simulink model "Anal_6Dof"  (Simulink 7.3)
settings: Solver=ode45  StartTime=0.0  StopTime=500  RelTol=1e-3
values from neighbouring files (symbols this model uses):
  calfa = cos(alfa0*d2r)    [run.m]
  d2r = pi/180    (= 0.0174532925199)    [run.m]
  klr = [0.82083770557  -0.70145835124   0.75722294555   0.32691190448   0.14993771995;        0.55253708187   0.66141640307  -0.4963339086    0.20601876795  -0.07844376733]    [run.m]
  kls = [0.23009875115  -1.3857134134    0.5565800989    0.03843893525  0.1360972015;        0.22658853965   0.3268097242   -0.0904376422    0.0272194403  -0.00768778705]    [run.m]
  r2d = 180/pi    (= 57.2957795131)    [Pl.m]    (also in run.m)
  salfa = sin(alfa0*d2r)    [run.m]
  Thet0 = 43    [run.m]
  V0 = 18640    [run.m]
undefined symbols (not defined in the file or in its folder): A6d, B6d, C6d, D6d, KJmix, KSmix

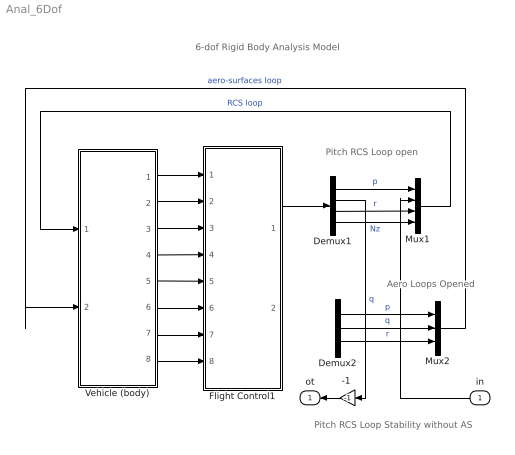
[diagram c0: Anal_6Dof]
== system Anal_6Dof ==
  note: 6-dof Rigid Body Analysis Model
  note: Pitch RCS Loop open
  note: Aero Loops Opened
  note: Pitch RCS Loop Stability without AS
  in : Inport  OutDataType=sfix(16)  OutScaling=2^0
  "-1 " : Gain  Gain=-1  ParameterDataType=sfix(16)  ParameterScaling=2^0  OutDataType=sfix(16)  OutScaling=2^0
  Demux1 : Demux
  Demux2 : Demux  Outputs=3
  Flight Control1 : Subsystem
  Mux1 : Mux
  Mux2 : Mux  Inputs=3
  Vehicle (body) : Subsystem
  ot : Outport  OutDataType=sfix(16)  OutScaling=2^0
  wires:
  Mux2/1 -> Vehicle (body)/2(Aer_pqr)  "aero-surfaces loop"
  Vehicle (body)/2(p) -> Flight Control1/2(pb)
  Vehicle (body)/3(r) -> Flight Control1/3(rb)
  Vehicle (body)/6(q) -> Flight Control1/6(q)
  Vehicle (body)/5(thet) -> Flight Control1/5(thet)
  Vehicle (body)/7(alf) -> Flight Control1/7(alfa)
  Vehicle (body)/4(bet) -> Flight Control1/4(beta)
  Vehicle (body)/1(phi) -> Flight Control1/1(phi)
  Vehicle (body)/8(Nz) -> Flight Control1/8(Nz)
  "-1 "/1 -> ot/1
  Mux1/1 -> Vehicle (body)/1(Jet_pqr)  "RCS loop"
  Demux1/4 -> Mux1/4  "Nz"
  Demux1/3 -> Mux1/3  "r"
  Demux1/1 -> Mux1/1  "p"
  Demux2/1 -> Mux2/1  "p"
  Demux2/3 -> Mux2/3  "r"
  Flight Control1/1(Jet_pqr) -> Demux1/1
  Demux2/2 -> Mux2/2  "q"
  Demux1/2 -> "-1 "/1  "q"
  in/1 -> Mux1/2

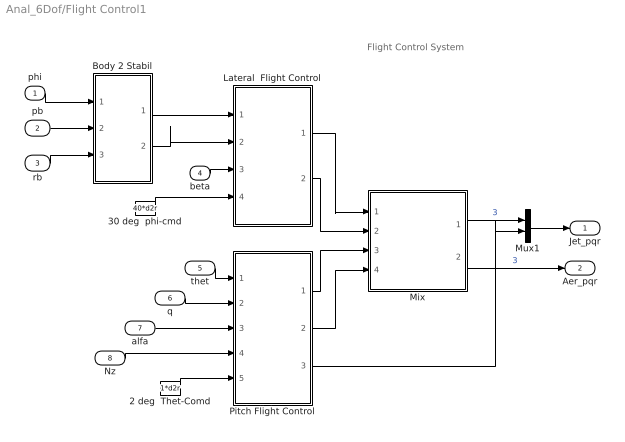
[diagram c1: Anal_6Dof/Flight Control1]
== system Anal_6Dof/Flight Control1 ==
  note: Flight Control System
  phi : Inport  OutDataType=sfix(16)  OutScaling=2^0
  pb : Inport  Port=2  OutDataType=sfix(16)  OutScaling=2^0
  rb : Inport  Port=3  OutDataType=sfix(16)  OutScaling=2^0
  beta : Inport  Port=4  OutDataType=sfix(16)  OutScaling=2^0
  thet : Inport  Port=5  OutDataType=sfix(16)  OutScaling=2^0
  q : Inport  Port=6  OutDataType=sfix(16)  OutScaling=2^0
  alfa : Inport  Port=7  OutDataType=sfix(16)  OutScaling=2^0
  Nz : Inport  Port=8  OutDataType=sfix(16)  OutScaling=2^0
  2 deg  Thet-Comd : Constant  Value=1*d2r  OutDataType=sfix(16)  OutScaling=2^0
  30 deg  phi-cmd : Constant  Value=40*d2r  OutDataType=sfix(16)  OutScaling=2^0
  Body 2 Stabil : Subsystem
  Lateral  Flight Control : Subsystem
  Mix : Subsystem
  Mux1 : Mux  Inputs=[3,1]
  Pitch Flight Control : Subsystem
  Jet_pqr : Outport  OutDataType=sfix(16)  OutScaling=2^0
  Aer_pqr : Outport  Port=2  OutDataType=sfix(16)  OutScaling=2^0
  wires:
  Lateral  Flight Control/1(rcs_PR) -> Mix/1(Rcs_PR)
  Lateral  Flight Control/2(aero_PR) -> Mix/2(Aer_PR)
  Pitch Flight Control/1(rcs_Q) -> Mix/3(Rcs_Q)
  Pitch Flight Control/2(aero_Q) -> Mix/4(Aer_Q)
  beta/1 -> Lateral  Flight Control/3(beta)
  Mix/2(Aer_pqr) -> Aer_pqr/1  "3"
  thet/1 -> Pitch Flight Control/1(thet)
  q/1 -> Pitch Flight Control/2(q)
  alfa/1 -> Pitch Flight Control/3(alf)
  Body 2 Stabil/2(r_s) -> Lateral  Flight Control/2(rs)
  Body 2 Stabil/1(p_s) -> Lateral  Flight Control/1(ps)
  rb/1 -> Body 2 Stabil/3(r_b)
  pb/1 -> Body 2 Stabil/2(p_b)
  phi/1 -> Body 2 Stabil/1(phi)
  Nz/1 -> Pitch Flight Control/4(Nz)
  Mix/1(Jet_pqr) -> Mux1/1  "3"
  2 deg  Thet-Comd/1 -> Pitch Flight Control/5(alf-cmd)
  30 deg  phi-cmd/1 -> Lateral  Flight Control/4(phi-cmd)
  Pitch Flight Control/3(Nzfb) -> Mux1/2
  Mux1/1 -> Jet_pqr/1

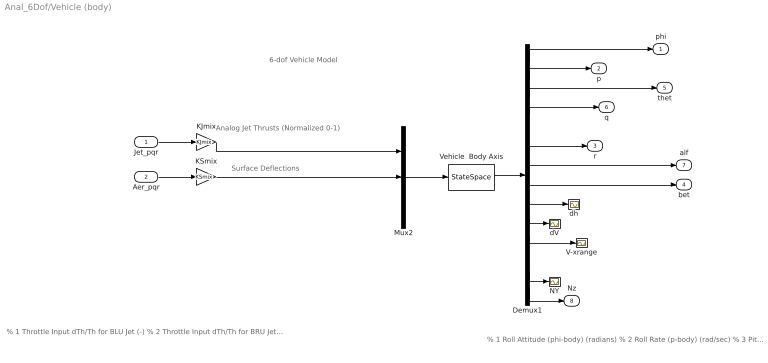
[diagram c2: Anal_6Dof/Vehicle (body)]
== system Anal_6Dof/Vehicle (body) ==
  note: 6-dof Vehicle Model
  note: % 1 Throttle Input dTh/Th for BLU Jet (-) % 2 Throttle Input dTh/Th for BRU Jet (-) % 3 Throttle Input dTh/Th for BLD Jet (-) % 4 Throttle Input dTh/Th for BRD Jet (-) % 5 Throttle Input dTh/Th for BL+Y Jet (-) % 6 Throttle Input dTh/Th for BR-Y Jet (-) % 7 Throttle Input dTh/Th for FU Jet (-) % 8 Throttle Input dTh/Th for FD Jet (-) % 9 Throttle Input dTh/Th for FL Jet (-) % 10 Throttle Input dTh/Th for FR Jet (-) % 11 Left Outbrd Elevon Deflection (radians) % 12 Left Inboard Elevon Deflection (radians) % 13 Right Inbrd Elevon Deflection (radians) % 14 Right Outbrd Elevon Deflection (radians) % 15 Vertical Rudder Deflection (radians) % 16 Gust Veloc, Azim-Elev Angles=(45,90) (deg)
  note: % 1 Roll Attitude (phi-body) (radians) % 2 Roll Rate (p-body) (rad/sec) % 3 Pitch Attitude (thet-bdy) (radians) % 4 Pitch Rate (q-body) (rad/sec) % 5 Yaw Attitude (psi-body) (radians) % 6 Yaw Rate (r-body) (rad/sec) % 7 Angle of attack, alfa, (radians) % 8 Angle of sideslip, beta, (radian) % 9 Change in Altitude, delta-h, (feet) % 10 Forward Acceleration (V-dot) (ft/sec) % 11 Cross Range Velocity (Vcr) (ft/sec) % 12 CG Acceleration along X axis, (ft/sec^2) % 13 CG Acceleration along Y axis, (ft/sec^2) % 14 CG Acceleration along Z axis, (ft/sec^2)
  note: Analog Jet Thrusts (Normalized 0-1)
  note: Surface Deflections
  Jet_pqr : Inport  OutDataType=sfix(16)  OutScaling=2^0
  Aer_pqr : Inport  Port=2  OutDataType=sfix(16)  OutScaling=2^0
  Demux1 : Demux  Outputs=14
  KJmix : Gain  Gain=KJmix  Multiplication=Matrix(K*u)  ParameterDataType=sfix(16)  ParameterScaling=2^0  OutDataType=sfix(16)  OutScaling=2^0
  KSmix : Gain  Gain=KSmix  Multiplication=Matrix(K*u)  ParameterDataType=sfix(16)  ParameterScaling=2^0  OutDataType=sfix(16)  OutScaling=2^0
  Mux2 : Mux  Inputs=[11, 5, 1]
  NY : Scope
  V-xrange : Scope
  Vehicle  Body Axis : StateSpace  A=A6d  B=B6d  C=C6d  D=D6d
  dV : Scope
  dh : Scope
  phi : Outport  OutDataType=sfix(16)  OutScaling=2^0
  p : Outport  Port=2  OutDataType=sfix(16)  OutScaling=2^0
  r : Outport  Port=3  OutDataType=sfix(16)  OutScaling=2^0
  bet : Outport  Port=4  OutDataType=sfix(16)  OutScaling=2^0
  thet : Outport  Port=5  OutDataType=sfix(16)  OutScaling=2^0
  q : Outport  Port=6  OutDataType=sfix(16)  OutScaling=2^0
  alf : Outport  Port=7  OutDataType=sfix(16)  OutScaling=2^0
  Nz : Outport  Port=8  OutDataType=sfix(16)  OutScaling=2^0
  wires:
  Demux1/11 -> V-xrange/1
  Demux1/13 -> NY/1
  Demux1/14 -> Nz/1
  Demux1/10 -> dV/1
  Demux1/9 -> dh/1
  Vehicle  Body Axis/1 -> Demux1/1
  Demux1/1 -> phi/1
  Demux1/3 -> thet/1
  Aer_pqr/1 -> KSmix/1
  Jet_pqr/1 -> KJmix/1
  Demux1/8 -> bet/1
  Demux1/7 -> alf/1
  Demux1/6 -> r/1
  Demux1/4 -> q/1
  Demux1/2 -> p/1
  KJmix/1 -> Mux2/1
  KSmix/1 -> Mux2/2
  Mux2/1 -> Vehicle  Body Axis/1

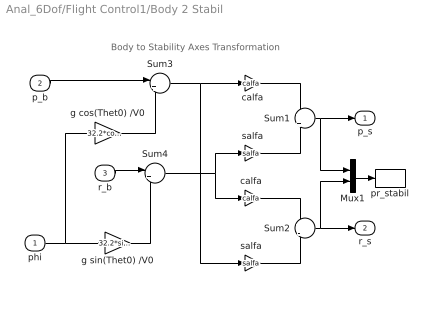
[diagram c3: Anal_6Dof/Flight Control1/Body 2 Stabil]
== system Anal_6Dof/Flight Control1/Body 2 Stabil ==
  note: Body to Stability Axes Transformation
  phi : Inport  OutDataType=sfix(16)  OutScaling=2^0
  p_b : Inport  Port=2  OutDataType=sfix(16)  OutScaling=2^0
  r_b : Inport  Port=3  OutDataType=sfix(16)  OutScaling=2^0
  Mux1 : Mux  Inputs=2
  Sum1 : Sum  Inputs=+|+  OutDataType=sfix(16)  OutScaling=2^0
  Sum2 : Sum  Inputs=+|-  OutDataType=sfix(16)  OutScaling=2^0
  Sum3 : Sum  Inputs=|++  OutDataType=sfix(16)  OutScaling=2^0
  Sum4 : Sum  Inputs=|+-  OutDataType=sfix(16)  OutScaling=2^0
  calfa : Gain  Gain=calfa  ParameterDataType=sfix(16)  ParameterScaling=2^0  OutDataType=sfix(16)  OutScaling=2^0
  "calfa " : Gain  Gain=calfa  ParameterDataType=sfix(16)  ParameterScaling=2^0  OutDataType=sfix(16)  OutScaling=2^0
  g cos(Thet0) /V0 : Gain  Gain=32.2*cos(Thet0*d2r)/V0  ParameterDataType=sfix(16)  ParameterScaling=2^0  OutDataType=sfix(16)  OutScaling=2^0
  g sin(Thet0) /V0 : Gain  Gain=32.2*sin(Thet0*d2r)/V0  ParameterDataType=sfix(16)  ParameterScaling=2^0  OutDataType=sfix(16)  OutScaling=2^0
  pr_stabil : ToWorkspace  VariableName=pr_st  SampleTime=-1  SaveFormat=Array
  salfa : Gain  Gain=salfa  ParameterDataType=sfix(16)  ParameterScaling=2^0  OutDataType=sfix(16)  OutScaling=2^0
  "salfa " : Gain  Gain=salfa  ParameterDataType=sfix(16)  ParameterScaling=2^0  OutDataType=sfix(16)  OutScaling=2^0
  p_s : Outport  OutDataType=sfix(16)  OutScaling=2^0
  r_s : Outport  Port=2  OutDataType=sfix(16)  OutScaling=2^0
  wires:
  Sum1/1 -> p_s/1, Mux1/1
  Sum2/1 -> r_s/1, Mux1/2
  p_b/1 -> Sum3/1
  r_b/1 -> Sum4/1
  g cos(Thet0) /V0/1 -> Sum3/2
  g sin(Thet0) /V0/1 -> Sum4/2
  phi/1 -> g cos(Thet0) /V0/1, g sin(Thet0) /V0/1
  Sum4/1 -> "calfa "/1, salfa/1
  Sum3/1 -> "salfa "/1, calfa/1
  calfa/1 -> Sum1/1
  salfa/1 -> Sum1/2
  "calfa "/1 -> Sum2/1
  "salfa "/1 -> Sum2/2
  Mux1/1 -> pr_stabil/1

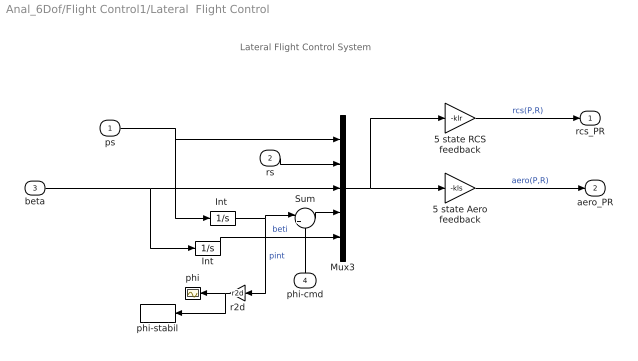
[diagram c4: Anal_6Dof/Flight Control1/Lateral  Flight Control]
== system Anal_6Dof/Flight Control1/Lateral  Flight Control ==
  note: Lateral Flight Control System
  ps : Inport  OutDataType=sfix(16)  OutScaling=2^0
  rs : Inport  Port=2  OutDataType=sfix(16)  OutScaling=2^0
  beta : Inport  Port=3  OutDataType=sfix(16)  OutScaling=2^0
  phi-cmd : Inport  Port=4  OutDataType=sfix(16)  OutScaling=2^0
  5 state Aero feedback : Gain  Gain=-kls  Multiplication=Matrix(K*u)  ParameterDataType=sfix(16)  ParameterScaling=2^0  OutDataType=sfix(16)  OutScaling=2^0
  5 state RCS feedback : Gain  Gain=-klr  Multiplication=Matrix(K*u)  ParameterDataType=sfix(16)  ParameterScaling=2^0  OutDataType=sfix(16)  OutScaling=2^0
  Int : Integrator
  "Int " : Integrator
  Mux3 : Mux  Inputs=5
  Sum : Sum  Inputs=|+-  OutDataType=sfix(16)  OutScaling=2^0
  phi : Scope
  phi-stabil : ToWorkspace  VariableName=phi_st  SampleTime=-1  SaveFormat=Array
  r2d : Gain  Gain=r2d  ParameterDataType=sfix(16)  ParameterScaling=2^0  OutDataType=sfix(16)  OutScaling=2^0
  rcs_PR : Outport  OutDataType=sfix(16)  OutScaling=2^0
  aero_PR : Outport  Port=2  OutDataType=sfix(16)  OutScaling=2^0
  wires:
  "Int "/1 -> Sum/1, r2d/1  "pint"
  Sum/1 -> Mux3/4
  Int/1 -> Mux3/5  "beti"
  beta/1 -> Int/1, Mux3/3
  ps/1 -> "Int "/1, Mux3/1
  Mux3/1 -> 5 state Aero feedback/1, 5 state RCS feedback/1
  rs/1 -> Mux3/2
  5 state RCS feedback/1 -> rcs_PR/1  "rcs(P,R)"
  5 state Aero feedback/1 -> aero_PR/1  "aero(P,R)"
  phi-cmd/1 -> Sum/2
  r2d/1 -> phi/1, phi-stabil/1

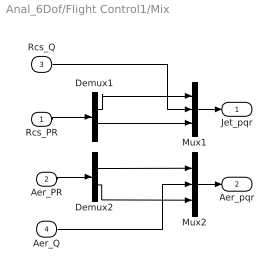
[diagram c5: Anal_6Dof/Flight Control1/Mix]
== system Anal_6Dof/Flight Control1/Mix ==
  Rcs_PR : Inport  OutDataType=sfix(16)  OutScaling=2^0
  Aer_PR : Inport  Port=2  OutDataType=sfix(16)  OutScaling=2^0
  Rcs_Q : Inport  Port=3  OutDataType=sfix(16)  OutScaling=2^0
  Aer_Q : Inport  Port=4  OutDataType=sfix(16)  OutScaling=2^0
  Demux1 : Demux  Outputs=2
  Demux2 : Demux  Outputs=2
  Mux1 : Mux  Inputs=3
  Mux2 : Mux  Inputs=3
  Jet_pqr : Outport  OutDataType=sfix(16)  OutScaling=2^0
  Aer_pqr : Outport  Port=2  OutDataType=sfix(16)  OutScaling=2^0
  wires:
  Demux1/1 -> Mux1/1
  Demux1/2 -> Mux1/3
  Demux2/1 -> Mux2/1
  Demux2/2 -> Mux2/3
  Mux1/1 -> Jet_pqr/1
  Rcs_PR/1 -> Demux1/1
  Aer_PR/1 -> Demux2/1
  Aer_Q/1 -> Mux2/2
  Mux2/1 -> Aer_pqr/1
  Rcs_Q/1 -> Mux1/2

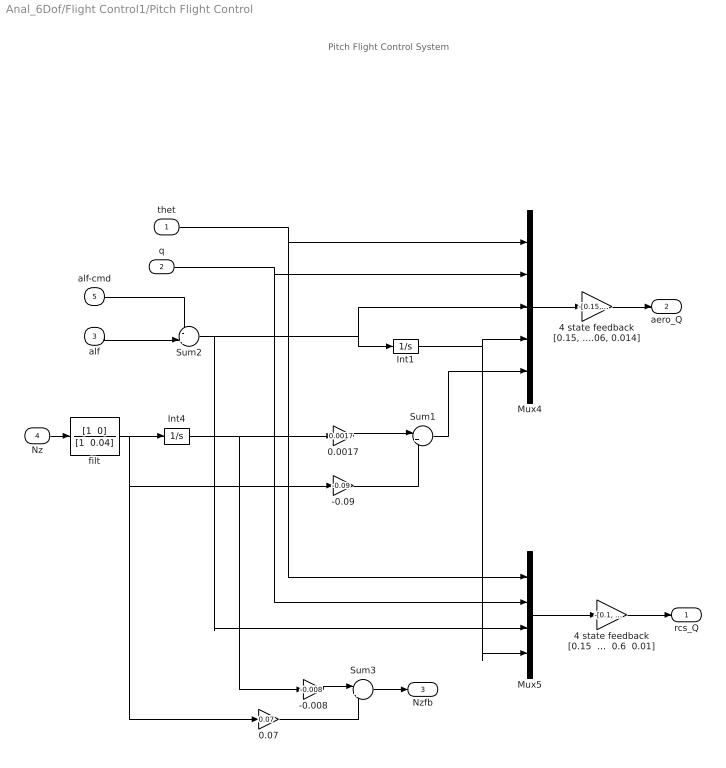
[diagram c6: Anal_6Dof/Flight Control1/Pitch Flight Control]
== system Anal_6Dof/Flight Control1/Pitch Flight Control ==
  note: Pitch Flight Control System
  thet : Inport  OutDataType=sfix(16)  OutScaling=2^0
  q : Inport  Port=2  OutDataType=sfix(16)  OutScaling=2^0
  alf : Inport  Port=3  OutDataType=sfix(16)  OutScaling=2^0
  Nz : Inport  Port=4  OutDataType=sfix(16)  OutScaling=2^0
  alf-cmd : Inport  Port=5  OutDataType=sfix(16)  OutScaling=2^0
  -0.008 : Gain  Gain=-0.008  ParameterDataType=sfix(16)  ParameterScaling=2^0  OutDataType=sfix(16)  OutScaling=2^0
  -0.09 : Gain  Gain=-0.09  ParameterDataType=sfix(16)  ParameterScaling=2^0  OutDataType=sfix(16)  OutScaling=2^0
  0.0017 : Gain  Gain=0.0017  ParameterDataType=sfix(16)  ParameterScaling=2^0  OutDataType=sfix(16)  OutScaling=2^0
  0.07 : Gain  Gain=0.07  ParameterDataType=sfix(16)  ParameterScaling=2^0  OutDataType=sfix(16)  OutScaling=2^0
  4 state feedback [0.15  1.8  0.6  0.01] : Gain  Gain="-[0.1,   1.8,   0.9,    0.01]"  Multiplication=Matrix(K*u)  ParameterDataType=sfix(16)  ParameterScaling=2^0  OutDataType=sfix(16)  OutScaling=2^0
  "4 state feedback [0.15, 2, 0.9, 0.06, 0.014]" : Gain  Gain="-[0.15,   2,   0.9,    0.06,   0.018]"  Multiplication=Matrix(K*u)  ParameterDataType=sfix(16)  ParameterScaling=2^0  OutDataType=sfix(16)  OutScaling=2^0
  Int1 : Integrator
  Int4 : Integrator
  Mux4 : Mux  Inputs=5
  Mux5 : Mux
  Sum1 : Sum  Inputs=|++  OutDataType=sfix(16)  OutScaling=2^0
  Sum2 : Sum  Inputs=-+|  OutDataType=sfix(16)  OutScaling=2^0
  Sum3 : Sum  Inputs=|++  OutDataType=sfix(16)  OutScaling=2^0
  filt : TransferFcn  Numerator="[1  0]"  Denominator="[1  0.04]"
  rcs_Q : Outport  OutDataType=sfix(16)  OutScaling=2^0
  aero_Q : Outport  Port=2  OutDataType=sfix(16)  OutScaling=2^0
  Nzfb : Outport  Port=3  OutDataType=sfix(16)  OutScaling=2^0
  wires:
  alf-cmd/1 -> Sum2/1
  alf/1 -> Sum2/2
  filt/1 -> 0.07/1, -0.09/1, Int4/1
  Int4/1 -> -0.008/1, 0.0017/1
  Sum3/1 -> Nzfb/1
  -0.008/1 -> Sum3/1
  0.07/1 -> Sum3/2
  4 state feedback [0.15  1.8  0.6  0.01]/1 -> rcs_Q/1
  Mux5/1 -> 4 state feedback [0.15  1.8  0.6  0.01]/1
  "4 state feedback [0.15, 2, 0.9, 0.06, 0.014]"/1 -> aero_Q/1
  Mux4/1 -> "4 state feedback [0.15, 2, 0.9, 0.06, 0.014]"/1
  Sum1/1 -> Mux4/5
  Nz/1 -> filt/1
  -0.09/1 -> Sum1/2
  0.0017/1 -> Sum1/1
  q/1 -> Mux5/2, Mux4/2
  thet/1 -> Mux5/1, Mux4/1
  Sum2/1 -> Mux5/3, Mux4/3, Int1/1
  Int1/1 -> Mux5/4, Mux4/4
